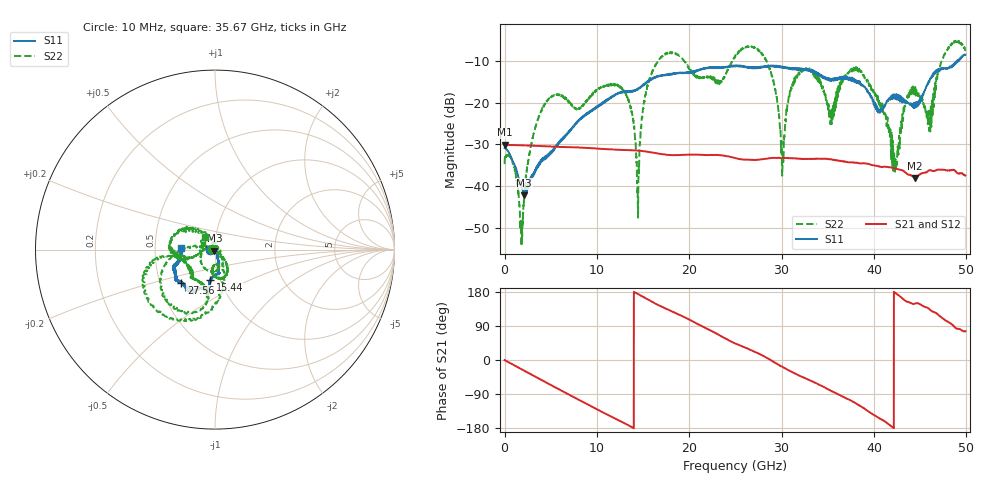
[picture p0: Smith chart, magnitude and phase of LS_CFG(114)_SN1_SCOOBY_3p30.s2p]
!Keysight Technologies,N5245B,MY58422026,A.13.80.08
!Date: Friday, March 20, 2020 00:02:59
!Correction: S11(Full 2 Port(1,2))
!S21(Full 2 Port(1,2))
!S12(Full 2 Port(1,2))
!S22(Full 2 Port(1,2))
!S2P File: Measurements: S11, S21, S12, S22:
# Hz S DB R 50.0
!freq dBS11 angS11 dBS21 angS21 dBS12 angS12 dBS22 angS22
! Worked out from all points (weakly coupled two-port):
!   4991 points, 10 MHz to 49.91 GHz, reference 50 ohm
!   highest |S21| = -30.11 dB at 20 MHz (marker M1); lowest = -38.1 dB at 44.46 GHz (marker M2)
!   lowest |S11| = -42.3 dB at 2.14 GHz (marker M3), VSWR 1.02, Z = 49.6 - j0.681 ohm
!   |S11| at or under -10 dB: start of sweep to 49.01 GHz; 49.04755 GHz to 49.10941 GHz (61.85 MHz wide, 0.126 % of centre); 49.18631 GHz to 49.21045 GHz (24.14 MHz wide, 0.0491 % of centre)
!   |S22| runs from -54.5 to -5.1 dB; largest |S21 - S12| = 0.00031
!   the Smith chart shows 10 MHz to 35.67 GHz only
!   S11 on the Smith chart (normalised r, x): 10 MHz: 0.94, -0.01; 15.44 GHz: 0.89, -0.32; 27.56 GHz: 0.65, -0.26; 35.67 GHz: 0.69, +0.01
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1e7  -30.91 -174.5  -30.12 -0.2  -30.10 -0.2  -34.77 177.3
2e7  -30.83 -178.6  -30.11 -0.3  -30.11 -0.4  -33.52 -178.8
2.14e9  -42.26 -117.1  -30.27 -28.4  -30.26 -28.3  -42.83 81.1
4.4e9  -32.92 -58.1  -30.49 -57.9  -30.47 -57.9  -20.30 -145.9
8.33e9  -23.88 -73.1  -30.84 -109.0  -30.83 -108.9  -21.04 -92.7
1.276e10  -17.53 -79.3  -31.37 -164.0  -31.37 -164.0  -16.75 -63.0
1.445e10  -16.81 -91.7  -31.54 174.0  -31.52 174.1  -46.36 -111.2
1.544e10  -15.23 -99.0  -31.81 160.6  -31.80 160.7  -16.43 174.4
1.665e10  -13.74 -99.0  -32.25 145.1  -32.24 145.2  -9.98 -157.3
2.496e10  -11.27 -125.3  -33.29 43.9  -33.28 44.2  -9.08 -167.9
2.756e10  -11.63 -135.4  -33.70 16.4  -33.70 16.8  -7.73 -110.0
3.011e10  -11.65 -145.6  -33.34 -17.9  -33.35 -17.7  -34.65 16.0
3.116e10  -11.84 -150.3  -33.39 -31.9  -33.38 -31.5  -15.61 140.2
3.328e10  -12.41 -160.3  -33.51 -56.1  -33.52 -55.7  -12.34 -175.3
3.567e10  -14.57 177.9  -33.75 -84.9  -33.70 -84.5  -20.91 127.8
3.816e10  -15.30 171.3  -34.47 -116.1  -34.42 -116.3  -11.58 -174.6
4.16e10  -19.09 100.2  -35.50 -169.7  -35.51 -169.6  -25.69 67.4
4.233e10  -18.35 100.0  -35.81 177.0  -35.84 177.0  -33.76 165.6
4.446e10  -20.16 48.8  -38.11 148.8  -38.11 149.2  -16.43 -7.2
4.6e10  -15.08 6.6  -36.23 134.2  -36.25 134.3  -24.53 112.1
4.771e10  -11.82 5.3  -36.18 105.1  -36.19 105.3  -8.15 -80.0
4.991e10  -8.48 -13.8  -37.50 76.0  -37.52 76.0  -7.38 -14.7
